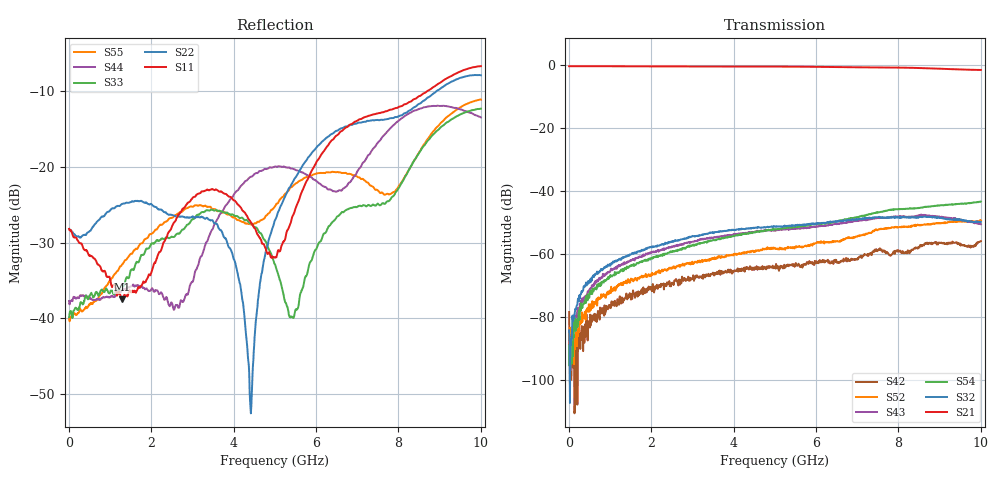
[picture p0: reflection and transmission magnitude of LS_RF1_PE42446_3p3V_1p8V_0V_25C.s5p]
! Created Wed Jan 31 17:13:26 2024
# ghz S ma R 50
! 5 Port Network Data from SP1.SP block
! freq  magS11  angS11  magS12  angS12  magS13  angS13  magS14  angS14
!  magS15  angS15
!  magS21  angS21  magS22  angS22  magS23  angS23
!  magS24  angS24  magS25  angS25
!  magS31  angS31  magS32  angS32
!  magS33  angS33  magS34  angS34  magS35  angS35
!  magS41  angS41
!  magS42  angS42  magS43  angS43  magS44  angS44  magS45  angS45
!  magS51  angS51  magS52  angS52  magS53  angS53  magS54  angS54
!  magS55  angS55
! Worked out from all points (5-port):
!   1000 points, 10 MHz to 10 GHz, reference 50 ohm
!   strongest paths, dB at 10 MHz, 2.51 GHz, 5.01 GHz, 7.51 GHz, 10 GHz:
!     S21: -0.5, -0.6, -0.7, -0.9, -1.7
!     S32: -84.4, -56.1, -51.4, -48.4, -49.9
!     S54: -95.4, -59.5, -52.4, -46.9, -43.5
!     S43: -89.6, -57.8, -52.7, -48.7, -50.7
!     S52: -84.5, -64.7, -58.3, -52.4, -49.5
!     S42: -78.6, -69.2, -64.6, -58.9, -56.0
!   lowest |S11| = -37.5 dB at 1.3 GHz (marker M1), VSWR 1.03, Z = 51.1 - j0.729 ohm
!   |S11| at or under -10 dB: start of sweep to 8.686 GHz
